FUNCTION_BLOCK FB_DO_IED_LD1_ATCC1_BndCtrChg EXTENDS FB_AcsiCommonControllableDataClass
VAR_INPUT
	mxVal: FB_AcsiDATypeAnalogueValue := (fc:=ACSI_FC_MX, TrgOp:=ACSI_TrgOp_dchg, bLinkResult:=THIS^.AddDataToContainer(ipData:=mxVal));
	q: FB_AcsiDATypeQuality := (fc:=ACSI_FC_MX, TrgOp:=ACSI_TrgOp_qchg, bLinkResult:=THIS^.AddDataToContainer(ipData:=q));
	t: FB_AcsiDATypeTimeStamp := (fc:=ACSI_FC_MX, bLinkResult:=THIS^.AddDataToContainer(ipData:=t));
	stSeld: FB_AcsiBATypeBOOLEAN := (fc:=ACSI_FC_MX, TrgOp:=ACSI_TrgOp_dchg, bLinkResult:=THIS^.AddDataToContainer(ipData:=stSeld));
	persistent_: FB_AcsiBATypeBOOLEAN := (sObjectName:='persistent', fc:=ACSI_FC_CF, TrgOp:=ACSI_TrgOp_dchg, bLinkResult:=THIS^.AddDataToContainer(ipData:=persistent_));
	ctlModel: FB_AcsiDATypeCtlModels := (fc:=ACSI_FC_CF, TrgOp:=ACSI_TrgOp_dchg, eValue:=E_AcsiCtlModels.SBOWithEnhancedSecurity, bLinkResult:=THIS^.AddDataToContainer(ipData:=ctlModel));
	sboTimeout: FB_AcsiBATypeINT32U := (fc:=ACSI_FC_CF, TrgOp:=ACSI_TrgOp_dchg, nValue:=30000, bLinkResult:=THIS^.AddDataToContainer(ipData:=sboTimeout));
	sboClass: FB_AcsiDATypeSboClasses := (fc:=ACSI_FC_CF, TrgOp:=ACSI_TrgOp_dchg, eValue:=E_AcsiSboClasses.OperateOnce, bLinkResult:=THIS^.AddDataToContainer(ipData:=sboClass));
	operTimeout: FB_AcsiBATypeINT32U := (fc:=ACSI_FC_CF, TrgOp:=ACSI_TrgOp_dchg, nValue:=30000, bLinkResult:=THIS^.AddDataToContainer(ipData:=operTimeout));
	Oper: FB_AcsiCDC_Oper_CODEDENUM := (fc:=ACSI_FC_CO, bLinkResult:=THIS^.AddDataToContainer(ipData:=Oper));
	SBOw: FB_AcsiCDC_SBOw_CODEDENUM := (fc:=ACSI_FC_CO, bLinkResult:=THIS^.AddDataToContainer(ipData:=SBOw));
	Cancel: FB_AcsiCDC_Cancel_CODEDENUM := (fc:=ACSI_FC_CO, bLinkResult:=THIS^.AddDataToContainer(ipData:=Cancel));
	
	fbControl: FB_SboControl := (ipCtrl:=THIS^.AddServerJob(ipEvent:=fbControl, ipCompletion:=fbControl), eType:=E_AcsiCDCType.BAC, ipBehVal:=fbIED.IEDLD1.ATCC1.Beh.stVal);
END_VAR
VAR
END_VAR

END_FUNCTION_BLOCK
